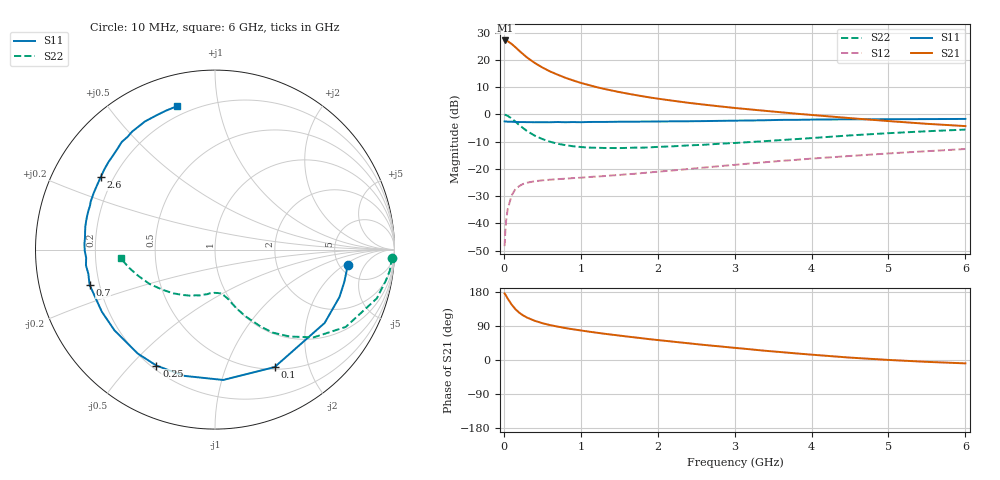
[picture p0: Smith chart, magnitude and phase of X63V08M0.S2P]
! SIEMENS Small Signal Semiconductors
! BFP193W
! Si NPN RF Bipolar Junction Transistor in SOT343
! VCE = 3 V  IC = 8 mA
! Common Emitter S-Parameters:  April 1994
# GHz  S  MA  R  50
!  f  S11  S21  S12  S22
! GHz  MAG  ANG  MAG  ANG  MAG  ANG  MAG  ANG
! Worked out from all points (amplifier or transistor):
!   40 points, 10 MHz to 6 GHz, reference 50 ohm
!   highest |S21| = 27.2 dB at 20 MHz (marker M1)
!   |S21| within 3 dB of that: start of sweep to 170.2 MHz
!   unconditionally stable (mu >= 1): 1.427 GHz to 4.157 GHz
!   at 200 MHz: K = 0.19, MSG = 24.9 dB, |S12| = -26.3 dB
!   at 1.5 GHz: K = 1.03, MAG = 14.2 dB, |S12| = -22.2 dB
!   at 6 GHz: K = 0.92, MSG = 4.2 dB, |S12| = -12.7 dB
!   lowest NFmin = 1.25 dB at 450 MHz
!   S11 on the Smith chart (normalised r, x): 10 MHz: 5.88, -2.33; 100 MHz: 0.53, -1.50; 250 MHz: 0.22, -0.59; 700 MHz: 0.16, -0.13; 2.6 GHz: 0.15, +0.28; 6 GHz: 0.15, +0.76
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0.01  0.7445 -6.8  22.84 175.5  0.0038 88.0  0.9873 -2.6
0.02  0.7426 -14.0  22.84 172.7  0.0075 82.4  0.9804 -7.0
0.03  0.7422 -20.8  22.7 169.1  0.0112 80.5  0.9675 -10.3
0.05  0.735 -33.8  22.1 162.0  0.0182 75.0  0.9415 -16.8
0.1  0.734 -63.1  19.76 146.7  0.0322 61.0  0.8463 -30.6
0.15  0.7278 -86.4  17.2 134.2  0.0424 50.8  0.7362 -41.6
0.2  0.7242 -103.8  14.76 124.8  0.0483 44.1  0.639 -49.3
0.25  0.7241 -116.8  12.82 117.8  0.0528 38.8  0.5621 -55.3
0.3  0.7215 -126.6  11.15 112.1  0.0556 35.5  0.4966 -59.4
0.4  0.7185 -141.2  8.854 103.6  0.0592 31.1  0.4089 -65.4
0.5  0.7193 -151.3  7.289 97.2  0.0615 29.1  0.3531 -69.5
0.6  0.7182 -158.4  6.164 92.2  0.0632 28.4  0.3154 -72.5
0.7  0.7255 -164.3  5.369 88.1  0.0647 28.4  0.2891 -74.6
0.9  0.7242 -173.1  4.213 81.0  0.0677 29.2  0.26 -79.0
1.1  0.7261 -179.6  3.477 75.0  0.0706 30.7  0.2458 -82.8
1.5  0.7339 169.8  2.575 64.5  0.0773 35.1  0.2407 -90.8
2.2  0.7458 155.0  1.782 48.4  0.0937 41.0  0.2596 -104.7
2.6  0.7541 147.6  1.515 39.9  0.1055 43.1  0.2769 -113.1
3.2  0.7732 137.3  1.236 28.3  0.1255 44.1  0.3109 -125.6
4.5  0.8136 118.7  0.855 6.3  0.1725 41.2  0.412 -152.3
5.5  0.8208 109.5  0.672 -4.9  0.211 36.6  0.4909 -168.3
6  0.8263 105.0  0.61 -8.9  0.2316 34.2  0.5265 -174.6
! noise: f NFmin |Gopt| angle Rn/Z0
0.45  1.25  0.23  133  0.12
0.9  1.3  0.35  156  0.11
1.8  2  0.55  -155  0.13
